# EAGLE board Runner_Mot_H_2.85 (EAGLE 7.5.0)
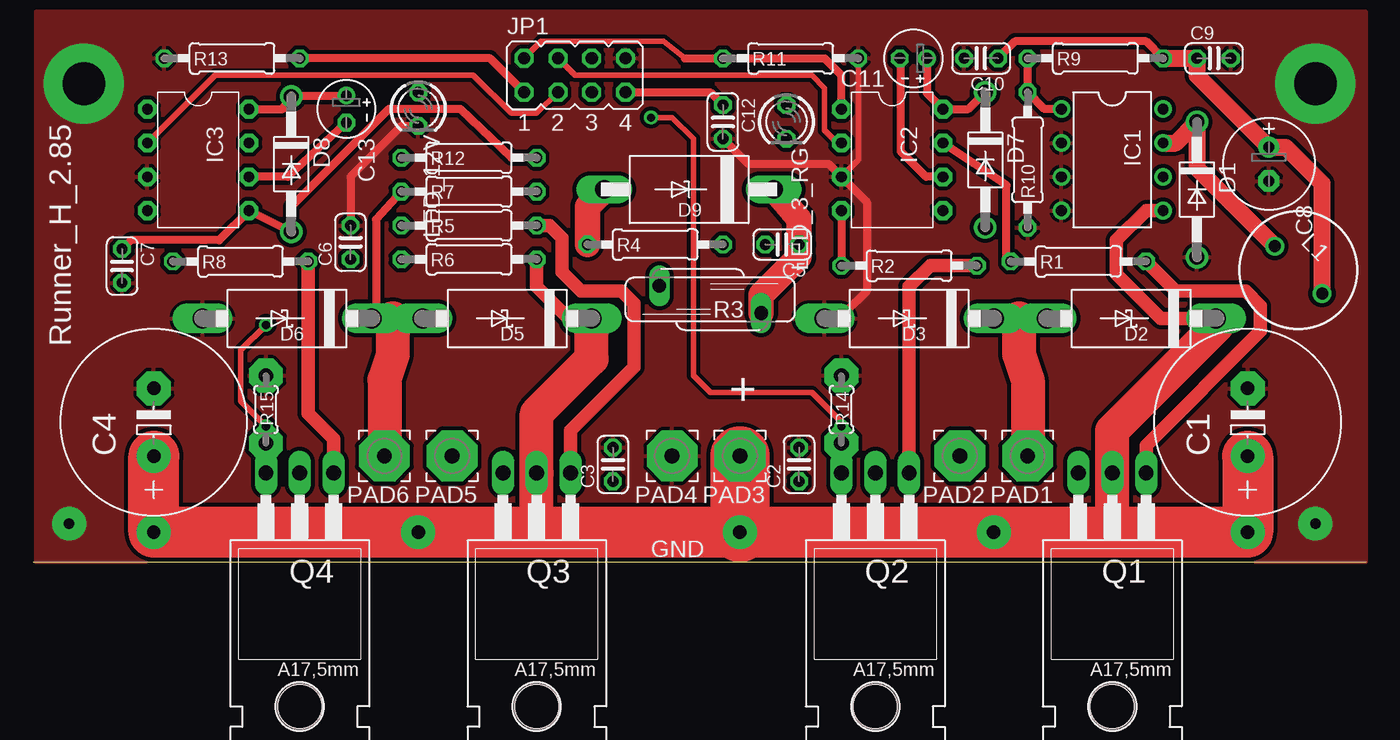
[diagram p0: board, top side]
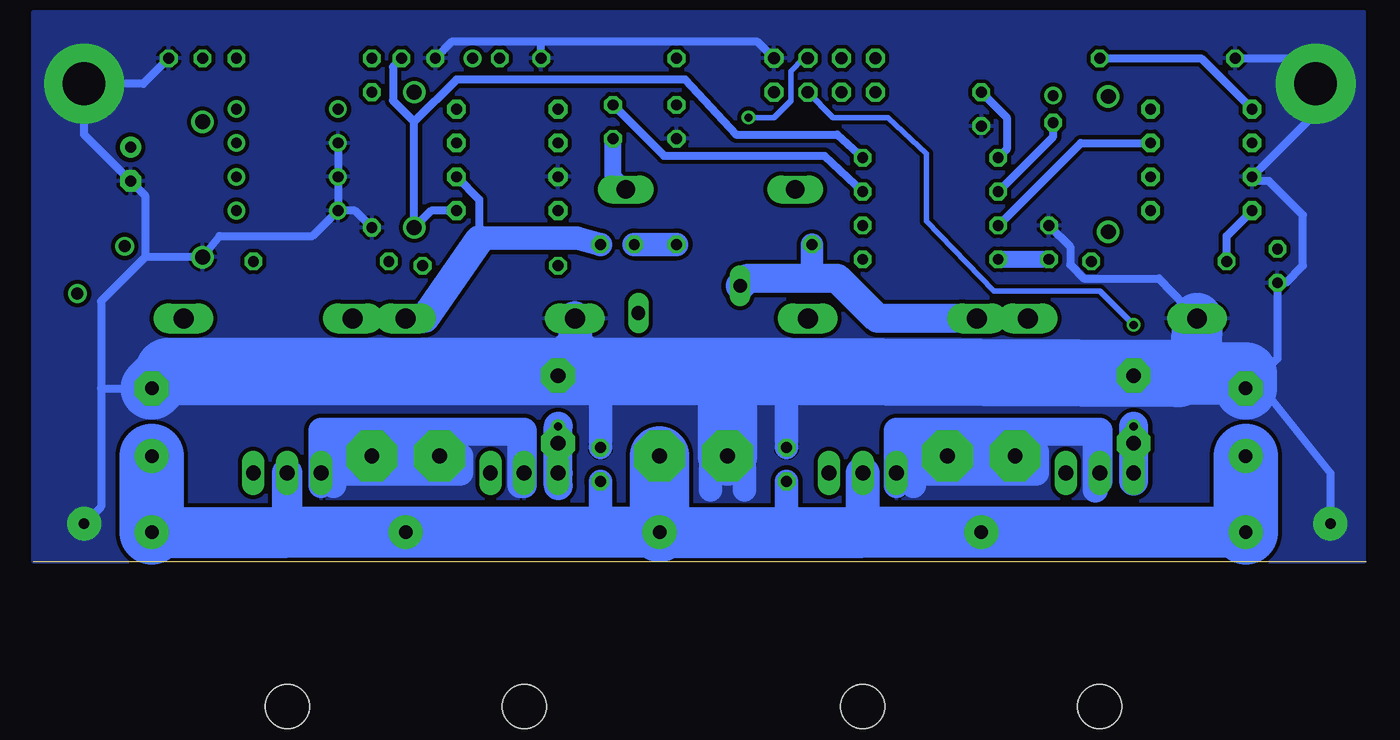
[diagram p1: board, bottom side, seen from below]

Size 100 x 0 mm. Coordinates in mm from the lower left corner, seen from the top.
Outline: 0,0 100,0
Copper layers (1*16): Top 0.035mm / dielectric 1.5mm / Bottom 0.035mm
Design rules "default *": minimum track width 10mil, minimum drill 24mil, track to track 12mil, track to pad 12mil, pad to pad 8mil, via to via 8mil, smd to smd 8mil, copper to edge 0mil, drill to drill 8mil, minimum pad ring 10mil, minimum via ring 8mil, stop-mask expansion 0mil, vias tented up to drill 0mil, thermal gap 10mil

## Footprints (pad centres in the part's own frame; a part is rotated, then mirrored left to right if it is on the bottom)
E5-13 = drill 1.016 pad 2.54: + -2.54,0 | drill 1.016 pad 2.54 octagon: - 2.54,0
C025-024X044 = drill 0.813 octagon: 1 -1.27,0; 2 1.27,0
E2,5-7 = drill 0.813 pad 1.6: + -1.27,0 | drill 0.813 pad 1.6 octagon: - 1.27,0
E2-4 = drill 0.813 pad 1.27: + -1.016,0 | drill 0.813 pad 1.27 octagon: - 1.016,0
DO41-10 = drill 1.118: A 5.08,0; C -5.08,0
DO201T15 = drill 1.499 long: A 6.35,0; C -6.35,0
CB429-17 = drill 1.397 long: A 6.35,0; C -6.35,0
DIL08 = drill 0.813 pad 1.27: 1 -3.81,-3.81; 2 -1.27,-3.81; 3 1.27,-3.81; 4 3.81,-3.81; 5 3.81,3.81; 6 1.27,3.81; 7 -1.27,3.81; 8 -3.81,3.81
IRF_DIL08 = drill 0.813 pad 1.397 octagon: 1 -3.81,-3.81; 2 -1.27,-3.81; 3 1.27,-3.81; 4 3.81,-3.81; 5 3.81,3.81; 6 1.27,3.81; 7 -1.27,3.81; 8 -3.81,3.81
JP4Q = drill 0.914 octagon: 1 -3.81,-1.27; 2 -3.81,1.27; 3 -1.27,-1.27; 4 -1.27,1.27; 5 1.27,-1.27; 6 1.27,1.27; 7 3.81,-1.27; 8 3.81,1.27
6000-XXXX-RC = drill 0.9 pad 1.422: 1 -2.5,0; 2 2.5,0
LED3MM = drill 0.813 octagon: A -1.27,0; K 1.27,0
3,81/1,1 = drill 1.118 pad 3.81 octagon: 1 0,0
TO220BH = drill 1.118 long: D 0,-6.35; G -2.54,-6.35; S 2.54,-6.35 | hole 3.302: 0,11.176
0207/10 = drill 0.813 octagon: 1 -5.08,0; 2 5.08,0
S10K40 = drill 1.016 long: 1 -1.016,-3.81; 2 1.016,3.81
0204/5 = drill 1.1 pad 2.54 octagon: 1 -2.54,0; 2 2.54,0

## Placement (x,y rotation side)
C1  RAD FR 680/50  [E5-13]  91.11,10.47 90 top  (outside the outline)
C2  100nF  [C025-024X044]  57.45,7.3 90 top  (outside the outline)
C3  100nF  [C025-024X044]  43.48,7.3 90 top  (outside the outline)
C4  RAD FR 680/50  [E5-13]  9.04,10.47 90 top  (outside the outline)
C5  100nF  [C025-024X044]  56.18,23.81 180 top  (outside the outline)
C6  100nF  [C025-024X044]  23.8,23.97 90 top  (outside the outline)
C7  100nF  [C025-024X044]  6.66,22.2 270 top  (outside the outline)
C8  220u/16V  [E2,5-7]  92.7,29.84 270 top  (outside the outline)
C9  100nF  [C025-024X044]  88.57,37.78 0 top  (outside the outline)
C10  100nF  [C025-024X044]  71.11,37.78 180 top  (outside the outline)
C11  4u7  [E2-4]  66.03,37.78 180 top  (outside the outline)
C12  100nF  [C025-024X044]  51.74,33.02 270 top  (outside the outline)
C13  4u7  [E2-4]  23.48,33.97 270 top  (outside the outline)
D1  1N5819  [DO41-10]  87.3,27.94 270 top  (outside the outline)
D2  1.5KE51A  [DO201T15]  82.38,18.25 180 top  (outside the outline)
D3  1.5KE51A  [DO201T15]  65.71,18.25 180 top  (outside the outline)
D5  1.5KE51A  [DO201T15]  35.55,18.25 180 top  (outside the outline)
D6  1.5KE51A  [DO201T15]  19.04,18.25 180 top  (outside the outline)
D7  SF18G  [DO41-10]  71.42,30.16 270 top  (outside the outline)
D8  SF18G  [DO41-10]  19.36,29.84 270 top  (outside the outline)
D9  1.5KE51CA  [CB429-17]  49.2,27.94 180 top  (outside the outline)
IC1  LM2574HVN-ADJ  [DIL08]  80.95,30.16 270 top  (outside the outline)
IC2  IRF_IR2184  [IRF_DIL08]  64.44,30.16 270 top  (outside the outline)
IC3  IRF_IR2184  [IRF_DIL08]  12.37,30.16 270 top  (outside the outline)
JP1  PWM_INP  [JP4Q]  40.63,36.51 0 top  (outside the outline)
L1  220uH  [6000-XXXX-RC]  94.92,21.9 315 top  (outside the outline)
LED_3_RG  PWM_LED  [LED3MM]  56.5,33.02 270 top  (outside the outline)
LED_12V  Power  [LED3MM]  28.88,33.97 270 top  (outside the outline)
PAD1  Motor_A  [3,81/1,1]  74.6,7.93 180 top  (outside the outline)
PAD2  Motor_A  [3,81/1,1]  69.52,7.93 180 top  (outside the outline)
PAD3  36V-45V  [3,81/1,1]  53.01,7.93 180 top  (outside the outline)
PAD4  GND  [3,81/1,1]  47.93,7.93 180 top  (outside the outline)
PAD5  Motor_B  [3,81/1,1]  31.42,7.93 180 top  (outside the outline)
PAD6  Motor_B  [3,81/1,1]  26.34,7.93 180 top  (outside the outline)
Q1  IRFB 4110  [TO220BH]  80.95,0.31 180 top
Q2  IRFB 4110  [TO220BH]  63.17,0.31 180 top
Q3  IRFB 4110  [TO220BH]  37.77,0.31 180 top
Q4  IRFB 4110  [TO220BH]  19.99,0.31 180 top
R1  4R7  [0207/10]  78.41,22.54 0 top  (outside the outline)
R2  4R7  [0207/10]  65.71,22.22 0 top  (outside the outline)
R3  Varistor 45V  [S10K40]  50.79,19.68 90 top  (outside the outline)
R4  0.47-1 Ohm  [0207/10]  46.66,23.81 0 top  (outside the outline)
R5  4R7  [0207/10]  32.69,25.24 0 top  (outside the outline)
R6  0.47-1 Ohm  [0207/10]  32.69,22.7 0 top  (outside the outline)
R7  4k7  [0207/10]  32.69,27.78 0 top  (outside the outline)
R8  4R7  [0207/10]  15.54,22.54 0 top  (outside the outline)
R9  18k  [0207/10]  79.68,37.78 0 top  (outside the outline)
R10  1k8  [0207/10]  74.6,30.16 90 top  (outside the outline)
R11  100k  [0207/10]  56.82,37.78 0 top  (outside the outline)
R12  4k7  [0207/10]  32.69,30.32 0 top  (outside the outline)
R13  100k  [0207/10]  14.91,37.78 0 top  (outside the outline)
R14  0.01  [0204/5]  60.63,11.42 270 top  (outside the outline)
R15  0.01  [0204/5]  17.45,11.42 270 top  (outside the outline)

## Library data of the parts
C1-C13 L1 = rcl
D1-D3 D5-D9 = diode
IC1-IC3 R3 = Runner_Mot_H_2.84x_doppelt
JP1 = jumper
LED_3_RG LED_12V = led
PAD1-PAD6 = wirepad
Q1-Q4 = transistor-power
R1 R2 R4-R13 = rcl_2
R14 R15 = resistor

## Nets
GND: C1.- C2.2 C3.2 C4.- C6.2 C7.2 C8.- C9.2 C10.2 C12.2 D1.A D3.A D6.A IC1.2 IC1.3 IC1.4 IC2.3 IC3.3 JP1.8 LED_12V.K PAD4.1 R10.1 R11.2 R13.1 R14.1 R15.1
N$1: IC3.1 JP1.1 R13.2
N$2: IC2.1 JP1.2 R11.1
N$3: C5.1 C11.- D2.A D3.C D9.C IC2.6 LED_3_RG.K PAD1.1 PAD2.1 Q1.S Q2.D R3.1
N$4: C11.+ D7.C IC2.8
N$5: IC2.7 R1.1
N$6: Q1.G R1.2
N$7: IC2.4 R2.1
N$8: Q2.G R2.2
N$9: C13.- D5.A D6.C D9.A IC3.6 PAD5.1 PAD6.1 Q3.S Q4.D R3.2 R4.1 R7.1
N$10: C13.+ D8.C IC3.8
N$11: IC3.7 R5.1
N$12: Q3.G R5.2
N$13: IC3.4 R8.1
N$14: Q4.G R8.2
N$15: C6.1 R6.1
N$16: C5.2 R4.2
N$17: IC3.2 JP1.3
N$18: IC2.2 JP1.4
N$19: LED_3_RG.A R7.2
N$20: JP1.6 Q2.S R14.2
N$22: IC1.1 R9.1 R10.2
N$24: LED_12V.A R12.1
N$25: JP1.5 Q4.S R15.2
N$33: D1.C IC1.7 L1.1
VCC5: C12.1 JP1.7
VCC15: C7.1 C8.+ C9.1 C10.1 D7.A D8.A IC2.5 IC3.5 L1.2 R9.2 R12.2
VCC24: C1.+ C2.1 C3.1 C4.+ D2.C D5.C IC1.5 PAD3.1 Q1.D Q3.D R6.2

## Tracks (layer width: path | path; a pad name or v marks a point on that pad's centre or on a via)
GND  (via drill 0.8 pad 2.54, 3.2 pad 6)
  Top 0.406: R11.2 61.9,30.16 IC2.3
  Top 0.61: D3.A 60.95,18.73 62.53,20.32 62.53,26.98 IC2.3 59.68,29.84 53.64,29.84 C12.2 | LED_12V.K 27.61,32.7 23.8,28.89 C6.2
  Bottom 0.61: IC1.2 IC1.3 IC1.4 | IC1.4 79.05,24.44 86.03,24.44 D1.A 91.61,22.86 | 91.61,22.86 94.92,19.55 94.92,13.01 | 94.92,13.01 C1.- | R10.1 75.87,26.35 IC1.4 | D6.A 15.54,21.27 21.2,21.27 22.21,22.28 22.21,23.65 C6.2 | C4.- 14.91,13.01 | C4.- 7.77,13.01 2.69,6.66 v2.69,2.85 | 94.92,13.01 94.92,4.12 v96.19,2.85 | C10.2 68.57,39.05 61.9,39.05 | C4.- 6.66,15.23 C7.2 6.04,20.93 4.75,22.22 4.75,26.03 7.29,28.57 8.24,28.57 IC3.3 3.8,33.65 v3.8,35.87 5.7,37.78 R13.1 | R11.2 61.9,39.05 | 61.9,39.05 45.71,39.05 JP1.8 | 91.61,22.86 91.61,27.48 C8.- 96.19,32.06 v96.19,35.87 91.74,35.87 C9.2 | 47.93,12.69 47.93,11.74 49.2,10.47
  Bottom 1.778: C2.2 57.46,14.28 | C3.2 43.49,14.28 | 49.2,5.39 49.2,10.47 | 46.66,5.39 46.66,9.2
  Bottom 2.54: D3.A 59.36,15.55
  Bottom 3.81: 59.36,15.55 60.63,14.28 | D6.A 12.85,14.12
  Bottom 4.445: PAD4.1 47.93,12.69 49.2,13.96 49.2,14.28
  Bottom 4.699: C4.- 9.04,14.12 12.85,14.12 14.12,14.12 | C1.- 89.84,14.28
  Bottom 5.08: 14.12,14.12 43.49,14.28 49.2,14.28 57.46,14.28 60.63,14.28 89.84,14.28
  pour Bottom: 100,-0.01 100,41.27 0.18,41.27 0.18,-0.01
  pour Top: 100,-0.01 100,41.27 0.18,41.27 0.18,-0.01
N$1
  Top 0.61: JP1.1 34.28,37.78 R13.2
  Bottom 0.61: R13.2 12.37,37.78 IC3.1
N$2
  Top 0.406: JP1.2 38.09,39.05 47.29,39.05 48.88,37.78
  Top 0.61: 48.88,37.78 R11.1 59.36,37.78 60.63,36.51 IC2.1
N$3
  Top 0.61: IC2.6 66.98,28.89 65.08,30.79 65.08,37.71 C11.-
  Top 1.27: C5.1 57.46,22.86
  Top 1.93: 57.46,22.86 54.6,20 R3.1 | C5.1 57.46,25.71 D9.C
  Top 2.184: D3.C 73.97,18.25 D2.A
  Top 2.54: PAD1.1 74.6,13.65 73.97,15.55 73.97,18.25
  Bottom 0.61: IC2.6 66.54,27.18 66.54,24.15
  Bottom 1.27: 66.54,24.15 66.19,24.28 | D9.C 56.5,28.89 LED_3_RG.K
  Bottom 1.778: 66.19,24.28 59.2,24.28 C5.1
  Bottom 1.93: 78.41,5.71 Q1.S 78.41,7.93 | 78.41,7.93 78.41,9.84 74.6,9.84 | PAD1.1 74.6,9.84 | 74.6,9.84 69.52,9.84 | PAD2.1 69.52,9.84 | 69.52,9.84 63.17,9.84 Q2.D 63.17,5.71 | 78.41,7.93 67.93,7.93 67.93,6.66 77.46,6.66 | 77.46,6.66 77.46,5.71 | 77.46,6.66 77.46,9.68 63.49,9.68 63.49,5.71
  Bottom 2.184: D3.C 70.63,18.25 66.54,24.15
  pour Bottom: 62.85,10.15 78.73,10.15 78.73,4.76 62.85,4.76
N$4
  Top 0.61: D7.C 70.16,33.97 IC2.8 67.04,35.17 C11.+
N$5
  Top 0.61: R1.1 73.01,22.86 73.01,28.25 IC2.7
N$6
  Top 1.016: Q1.G 83.49,8.73 92.06,17.3 92.06,19.2 90.95,20.32 85.71,20.32 R1.2
N$7
  Top 0.61: IC2.4 R2.1
N$8
  Top 1.016: Q2.G 65.71,20.63 67.3,22.22 R2.2
N$9
  Top 0.61: C13.- 19.1,28.89 IC3.6 | R7.1 25.71,25.71 25.71,18.73 D6.C
  Top 1.93: R4.1 41.58,26.67 D9.A
  Top 2.184: D6.C 26.98,18.25 D5.A
  Top 2.54: PAD6.1 26.34,13.65 26.98,15.55 26.98,18.25
  Bottom 0.61: R7.1 23.48,31.9 C13.-
  Bottom 1.676: 41.58,21.27 R4.1
  Bottom 1.93: 35.23,5.71 Q3.S 35.23,9.84 31.42,9.84 | PAD5.1 31.42,9.84 | 31.42,9.84 26.34,9.84 | PAD6.1 26.34,9.84 | 26.34,9.84 19.99,9.84 Q4.D 19.99,6.03 | 33.96,5.71 33.96,8.25 24.75,8.25 24.75,6.66 33.96,6.66 | 34.28,6.66 33.96,6.66 | 33.96,6.66 33.96,9.68 20.31,9.68 20.31,5.39
  Bottom 2.184: D5.A 36.66,18.25 39.68,21.27 41.58,21.27 46.41,21.27 R3.2
  pour Bottom: 19.67,10.15 35.55,10.15 35.55,4.76 19.67,4.76
N$10
  Top 0.61: IC3.8 18.72,33.97 D8.C 23.42,34.92 C13.+
N$11
  Bottom 0.61: R5.1 21.42,31.43 IC3.7
N$12
  Top 1.016: R5.2 38.72,25.24 39.68,24.28 39.68,21.74 41.1,20.32 44.12,20.32 45.07,19.36 45.07,14.6 40.31,9.84 Q3.G
N$13
  Bottom 0.61: R8.1 10.46,24.44 IC3.4
N$14
  Top 1.016: Q4.G 22.53,9.2 20.62,11.11 R8.2
N$15
  Bottom 1.27: R6.1 C6.1
N$16
  Bottom 1.778: C5.2 R4.2
N$17
  Top 0.406: IC3.2 13.64,36.51 33.01,36.51 35.86,33.65 37.77,33.65 JP1.3
N$18
  Top 0.406: IC2.2 60.31,31.43 59.36,32.38 59.36,35.55 58.41,36.51 40.63,36.51 JP1.4
N$19
  Bottom 0.61: LED_3_RG.A 52.69,30.48 40.63,30.48 R7.2
N$20  (via drill 0.61)
  Top 0.406: v60.63,10.15 60.63,10.47 58.41,12.69 50.79,12.69 49.52,13.96 49.52,31.75 47.93,33.33 v46.34,33.33
  Bottom 0.406: JP1.6 42.21,37.78 43.17,36.82 43.17,34.6 44.44,33.33 v46.34,33.33
  Bottom 2.184: Q2.S R14.2 | 60.63,5.71 Q2.S | Q2.S v60.63,10.15
N$22
  Top 0.61: IC1.1 75.87,33.97 R10.2 R9.1
N$24
  Bottom 0.61: LED_12V.A 26.98,33.33 26.98,30.95 R12.1
N$25  (via drill 0.61)
  Top 0.406: v17.45,10.15 15.54,12.06 15.54,15.87 v17.45,17.78
  Bottom 0.406: v17.45,17.78 19.99,20.32 27.93,20.32 33.01,25.55 33.01,30.63 35.86,33.33 39.99,33.33 JP1.5
  Bottom 2.184: Q4.S R15.2 | 17.45,6.03 Q4.S | Q4.S v17.45,10.15
N$33
  Top 1.27: IC1.7 85.71,31.43 D1.C 87.3,29.52 L1.1
VCC5
  Top 0.61: JP1.7 50.79,35.24 C12.1
VCC15
  Top 0.61: C7.1 7.29,24.12 13.96,24.12 IC3.5 D8.A 19.35,26.67 26.66,33.97 32.06,33.97 35.86,30.32 R12.2 | R9.2 83.49,39.05 73.65,39.05 C10.1
  Top 1.27: L1.2 96.69,28.39 93.97,31.11 C8.+ 87.3,36.51 C9.1 R9.2
  Bottom 0.61: R12.2 39.68,32.06 47.29,32.06 51.1,36.19 68.25,36.19 71.43,33.02 | IC2.5 70.16,26.35 D7.A 71.43,33.02 | C10.1 73.01,37.14 73.01,34.6 71.43,33.02
VCC24  (via drill 1 pad 2.54)
  Top 1.016: D5.C 40.15,18.25 37.77,20.63 R6.2 | IC1.5 83.49,26.35 81.27,24.12 81.27,21.59 84.6,18.25 D2.C
  Top 1.27: 88.73,17.62 D2.C
  Top 1.778: 41.9,17.46 D5.C
  Top 2.54: 37.77,2.22 Q3.D 37.77,11.11 41.9,15.23 41.9,17.46 | 80.95,2.22 Q1.D 80.95,9.84 88.73,17.62
  Top 3.81: C1.+ v91.11,2.22 80.95,2.22 v53.01,2.22 37.77,2.22 v9.04,2.22 C4.+
  Top 4.445: v53.01,2.22 PAD3.1
  Bottom 1.778: C2.1 57.46,2.22 | C3.1 43.49,2.22
  Bottom 2.286: 80.95,2.22 Q1.D
  Bottom 2.54: 37.77,2.22 Q3.D | v91.11,2.22 90.47,2.85 89.84,2.22
  Bottom 3.81: v9.04,2.22 v28.88,2.22 37.77,2.22 43.49,2.22 v53.01,2.22 57.46,2.22 v72.06,2.22 80.95,2.22 89.84,2.22
  Bottom 4.445: PAD3.1 v53.01,2.22
  Bottom 4.826: C4.+ v9.04,2.22 | C1.+ v91.11,2.22

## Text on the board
tNames: Runner_H_2.85 | + | GND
